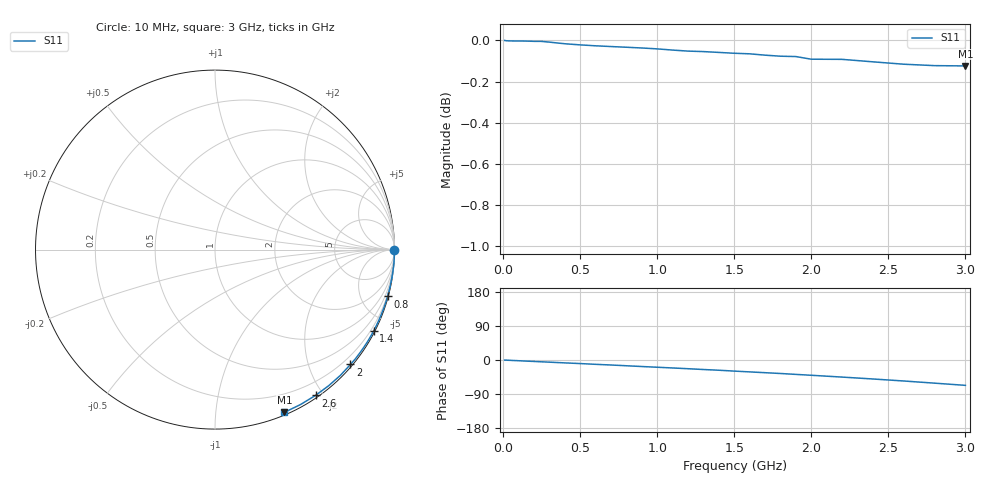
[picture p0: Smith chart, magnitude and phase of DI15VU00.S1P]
! SIEMENS Small Signal Semiconductors
! BAV99
! Silicon Switching Diode in SOT23
! VR = 15 V
! S-Parameters:  May  1995
# GHz  S  MA  R  50
!  f  S11
! GHz  MAG  ANG
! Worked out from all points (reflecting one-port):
!   30 points, 10 MHz to 3 GHz, reference 50 ohm
!   lowest |S11| = -0.1 dB at 3 GHz (marker M1), VSWR 140.24, Z = 1.17 - j75.7 ohm
!   phase of S11 starts at -0 deg and turns -67 deg over the sweep
!   S11 on the Smith chart (normalised r, x): 10 MHz: open; 800 MHz: 0.11, -7.49; 1.4 GHz: 0.06, -4.16; 2 GHz: 0.04, -2.72; 2.6 GHz: 0.03, -1.90; 3 GHz: 0.02, -1.51
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0.01  1 -0.2
0.05  0.9997 -1.0
0.1  0.9997 -1.9
0.15  0.9996 -2.9
0.2  0.9995 -3.8
0.25  0.9995 -4.8
0.3  0.9991 -5.7
0.4  0.9981 -7.6
0.5  0.9975 -9.4
0.6  0.997 -11.4
0.7  0.9966 -13.2
0.8  0.9962 -15.2
0.9  0.9958 -17.2
1  0.9953 -19.1
1.1  0.9946 -21.0
1.2  0.994 -23.0
1.3  0.9938 -25.1
1.4  0.9933 -27.0
1.5  0.9929 -29.3
1.6  0.9925 -31.4
1.8  0.9912 -35.6
1.9  0.991 -38.0
2  0.9896 -40.3
2.2  0.9895 -45.1
2.4  0.9881 -50.1
2.6  0.9868 -55.4
2.8  0.986 -61.1
3  0.9858 -66.9
